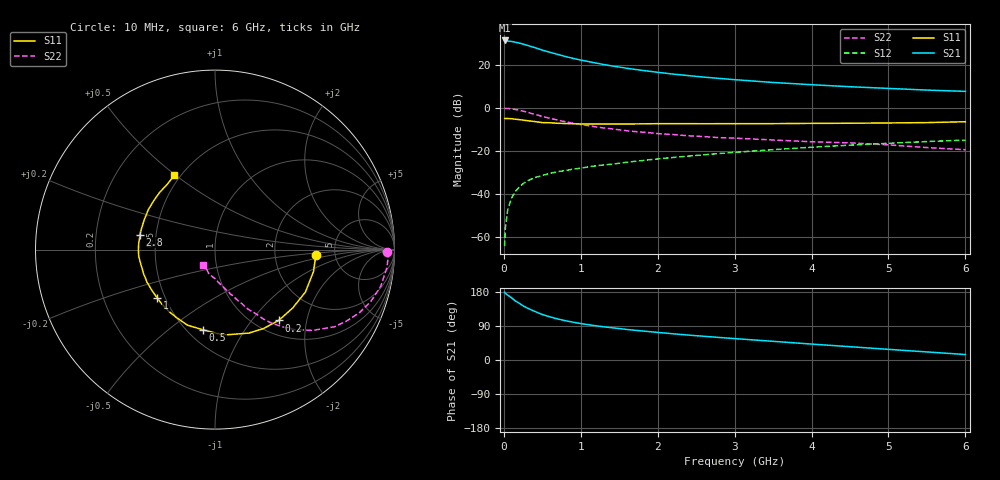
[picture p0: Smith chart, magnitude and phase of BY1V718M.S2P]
! SIEMENS Small Signal Semiconductors
! BFY420
! Si NPN RF SIEGET Grounded Emitter Transistor in MICRO-X
! VCE = 1.75 V  IC = 18 mA
! Common Emitter S-Parameters:  October  1996
# GHz  S  MA  R  50
!  f  S11  S21  S12  S22
! GHz  MAG  ANG  MAG  ANG  MAG  ANG  MAG  ANG
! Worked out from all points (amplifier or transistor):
!   36 points, 10 MHz to 6 GHz, reference 50 ohm
!   highest |S21| = 31.3 dB at 10 MHz (marker M1)
!   |S21| within 3 dB of that: start of sweep to 370.7 MHz
!   unconditionally stable (mu >= 1): start of sweep to 10.64 MHz; 1.994 GHz to end of sweep
!   at 250 MHz: K = 0.27, MSG = 32.5 dB, |S12| = -35.3 dB
!   at 1.4 GHz: K = 0.90, MSG = 22.9 dB, |S12| = -26.3 dB
!   at 6 GHz: K = 1.08, MAG = 9.6 dB, |S12| = -15.0 dB
!   S11 on the Smith chart (normalised r, x): 10 MHz: 3.55, -0.30; 200 MHz: 1.26, -1.38; 500 MHz: 0.60, -0.67; 1 GHz: 0.45, -0.30; 2.8 GHz: 0.41, +0.08; 6 GHz: 0.46, +0.50
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0.01  0.5627 -2.9  36.92 178.9  0.0006 99.4  0.96 -0.7
0.02  0.5613 -5.3  36.72 175.9  0.0016 91.0  0.9663 -2.1
0.1  0.5565 -25.2  35.03 164.2  0.0079 80.0  0.9458 -12.5
0.15  0.5413 -36.9  33.57 155.8  0.0113 74.4  0.915 -18.4
0.2  0.5309 -48.0  32.13 149.8  0.0143 72.0  0.8781 -23.6
0.25  0.5161 -58.5  30.4 143.0  0.0171 67.9  0.8332 -28.6
0.3  0.5019 -68.0  28.59 137.5  0.0197 64.8  0.792 -32.9
0.4  0.4783 -84.4  25.19 128.4  0.0236 61.0  0.705 -39.7
0.5  0.4517 -98.5  21.97 120.0  0.0266 59.0  0.6306 -45.0
0.6  0.4483 -110.0  19.58 113.8  0.0297 57.4  0.5681 -49.1
0.7  0.4352 -119.5  17.48 108.3  0.0325 55.9  0.5171 -52.4
0.8  0.4297 -127.2  15.62 103.7  0.0346 54.6  0.4725 -55.1
1  0.4197 -139.8  12.91 96.2  0.0393 54.8  0.4076 -58.6
1.1  0.4189 -146.2  11.91 93.1  0.0422 54.9  0.3821 -60.8
1.4  0.4188 -157.9  9.429 85.2  0.0486 55.2  0.3237 -64.7
1.6  0.4194 -165.4  8.297 80.5  0.0541 54.9  0.2922 -67.4
2.2  0.4268 -179.9  6.085 69.2  0.0697 53.4  0.2379 -73.8
2.8  0.4263 168.7  4.825 59.5  0.086 50.9  0.2018 -79.4
3.5  0.4278 156.9  3.884 49.3  0.1058 46.5  0.1778 -85.6
4.5  0.4368 141.5  3.092 35.1  0.1348 38.5  0.1524 -95.3
5.5  0.4518 125.6  2.583 21.3  0.1636 29.3  0.1184 -113.6
6  0.4731 118.5  2.409 14.4  0.177 24.4  0.1055 -127.7
